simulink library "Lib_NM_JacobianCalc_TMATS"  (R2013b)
settings: Solver=ode45  StartTime=0.0  StopTime=10.0  RelTol=1e-3
undefined symbols (not defined in the file or in its folder): N_Ind_M, N_Per_M

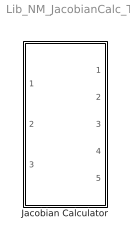
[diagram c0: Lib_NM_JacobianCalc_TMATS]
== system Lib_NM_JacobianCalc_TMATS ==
  Jacobian Calculator : Subsystem  TreatAsAtomicUnit=on

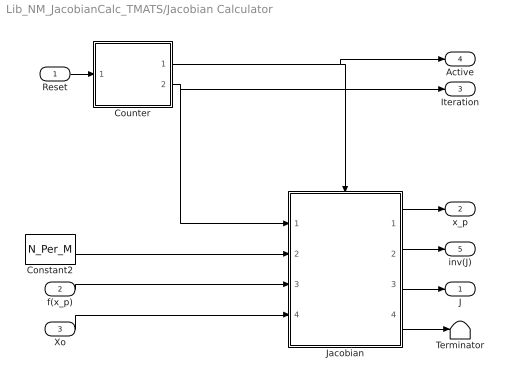
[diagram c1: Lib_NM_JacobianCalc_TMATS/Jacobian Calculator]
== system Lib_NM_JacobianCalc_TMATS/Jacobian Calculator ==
  Reset : Inport
  f(x_p) : Inport  Port=2
  Xo : Inport  Port=3
  Constant2 : Constant  Value=N_Per_M
  Counter : Subsystem
  Jacobian : Subsystem
  Terminator : Terminator
  J : Outport
  x_p : Outport  Port=2
  Iteration : Outport  Port=3
  Active : Outport  Port=4
  inv(J) : Outport  Port=5
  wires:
  f(x_p)/1 -> Jacobian/3(f(x_p))
  Constant2/1 -> Jacobian/2(Per)
  Jacobian/1(x_p) -> x_p/1
  Reset/1 -> Counter/1(Reset)
  Counter/1(Enable) -> Active/1, Jacobian/Enable
  Xo/1 -> Jacobian/4(Xo)
  Counter/2(Iteration) -> Iteration/1, Jacobian/1(Iteration)
  Jacobian/2(Inv(J)) -> inv(J)/1
  Jacobian/3(J) -> J/1
  Jacobian/4(y_State) -> Terminator/1

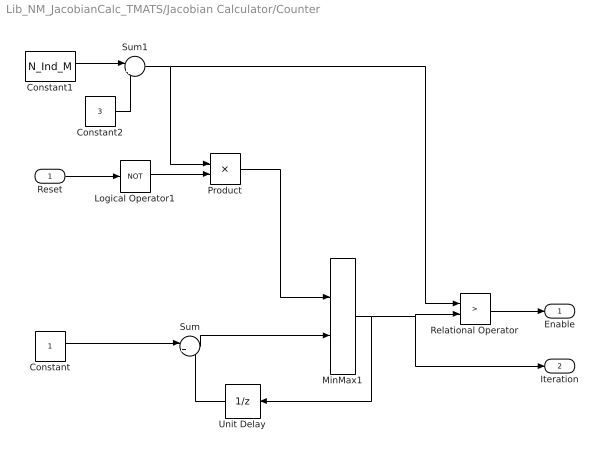
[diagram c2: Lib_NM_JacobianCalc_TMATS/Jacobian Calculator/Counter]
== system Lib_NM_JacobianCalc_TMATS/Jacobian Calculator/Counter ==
  Reset : Inport
  Constant : Constant
  Constant1 : Constant  Value=N_Ind_M
  Constant2 : Constant  Value=3
  Logical Operator1 : Logic  Operator=NOT  AllPortsSameDT=off  OutDataTypeStr=boolean
  MinMax1 : MinMax  Inputs=2
  Product : Product
  Relational Operator : RelationalOperator  Operator=>  OutDataTypeStr=boolean
  Sum : Sum  Inputs=|++
  Sum1 : Sum  Inputs=|++
  Unit Delay : UnitDelay  SampleTime=-1
  Enable : Outport
  Iteration : Outport  Port=2
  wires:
  Constant/1 -> Sum/1
  Product/1 -> MinMax1/1
  Sum/1 -> MinMax1/2
  Unit Delay/1 -> Sum/2
  MinMax1/1 -> Unit Delay/1, Iteration/1, Relational Operator/2
  Relational Operator/1 -> Enable/1
  Logical Operator1/1 -> Product/2
  Reset/1 -> Logical Operator1/1
  Sum1/1 -> Relational Operator/1, Product/1
  Constant2/1 -> Sum1/2
  Constant1/1 -> Sum1/1

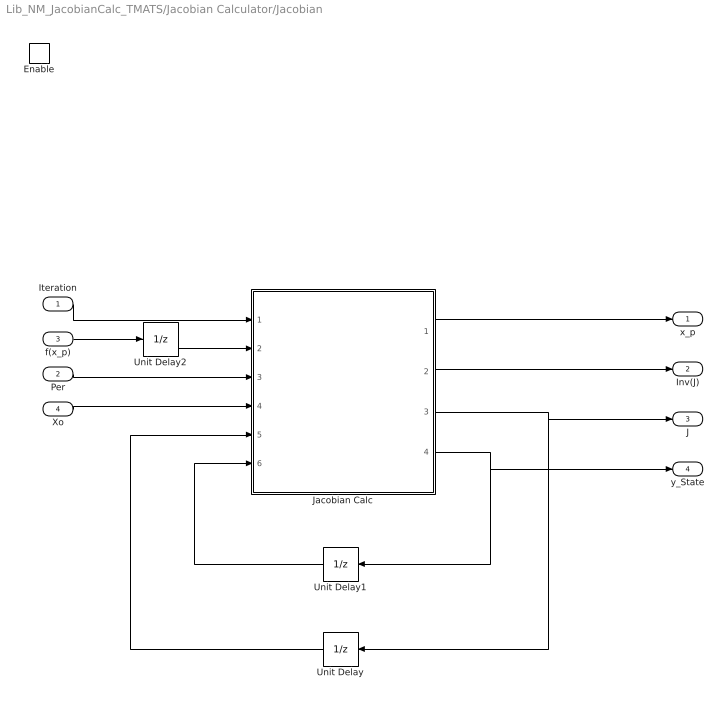
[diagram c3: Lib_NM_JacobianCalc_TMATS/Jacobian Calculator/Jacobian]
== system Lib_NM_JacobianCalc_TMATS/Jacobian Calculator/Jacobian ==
  Iteration : Inport
  Per : Inport  Port=2
  f(x_p) : Inport  Port=3
  Xo : Inport  Port=4
  Enable : EnablePort
  Jacobian Calc : MATLAB Function  TreatAsAtomicUnit=on
  Unit Delay : UnitDelay  InitialCondition=zeros(length(N_Per_M),length(N_Per_M))  SampleTime=-1
  Unit Delay1 : UnitDelay  InitialCondition=zeros(length(N_Per_M),length(N_Per_M)+1)  SampleTime=-1
  Unit Delay2 : UnitDelay  InitialCondition=zeros(length(N_Per_M),1)  SampleTime=-1
  x_p : Outport
  Inv(J) : Outport  Port=2
  J : Outport  Port=3
  y_State : Outport  Port=4
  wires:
  Jacobian Calc/1(XpOut) -> x_p/1
  Xo/1 -> Jacobian Calc/4(XoIn)
  Per/1 -> Jacobian Calc/3(PerIn)
  Iteration/1 -> Jacobian Calc/1(IterationIn)
  Jacobian Calc/3(JOut) -> Unit Delay/1, J/1
  Jacobian Calc/2(InvJOut) -> Inv(J)/1
  Unit Delay/1 -> Jacobian Calc/5(JStateIn)
  Jacobian Calc/4(y_StateOut) -> y_State/1, Unit Delay1/1
  Unit Delay1/1 -> Jacobian Calc/6(y_StateIn)
  f(x_p)/1 -> Unit Delay2/1
  Unit Delay2/1 -> Jacobian Calc/2(y_xpIn)
